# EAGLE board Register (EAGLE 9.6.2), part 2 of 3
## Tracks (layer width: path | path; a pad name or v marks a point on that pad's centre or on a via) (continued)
GND  (via drill 0.35) (continued)
  Bottom 0.152: 30.47,60.25 30.47,61.49 C82.2 30.47,61.67 30.47,73.23 C77.2 30.47,73.41 30.47,84.96 C75.2 31.91,85.09 32.07,85.25 32.07,87.78 30.47,89.38 30.47,96.16 C10.2 30.47,96.34 30.47,107.54 C53.2 30.65,107.72 30.65,108.79 | 30.47,60.25 v34.02,60.25 37.22,63.45 43.27,63.45 | 30.65,109.14 30.65,115.19 GND.1 | 30.65,109.14 30.65,108.79 | 30.65,109.14 v32.07,109.14 | 30.47,16.51 30.47,27.89 C48.2 | C74.2 18.73,27.89 C14.2 18.73,28.07 18.73,39.27 C18.2 18.73,39.45 C65.2 18.73,50.65 18.73,61.85 C60.2 18.73,62.03 18.73,65.88 19.84,66.99 19.84,71.12 18.73,72.23 18.73,73.23 C55.2 18.55,73.41 18.55,78.34 16.95,79.94 16.95,84.96 C11.2 16.78,85.14 16.78,96.16 C69.2 16.95,96.34 16.95,102.39 17.13,102.57 17.13,106.48 | 30.47,16.51 29.4,15.44 v21.76,15.44 20.33,15.44 19.27,16.51 C74.2 | 30.47,16.51 C28.2 | C74.2 | 17.13,106.48 10.95,106.48 9.48,107.95 C9.2 8.06,108.08 8.15,107.99 8.15,100.53 7,99.38 7,96.88 C1.2 7,96.7 7,85.5 C3.2 7,85.32 7,74.12 C5.2 7,73.94 7,62.56 C7.2 | 17.13,106.48 17.49,106.48 18.55,107.54 C19.2 | v4.69,109.64 5.52,110.47 17.23,110.47 18.73,108.98 C19.2 | 7,62.33 7,62.38 C7.2 | 7,62.33 7,61.85 | 7,61.85 7,51.18 C2.2 7,51 7,39.8 C4.2 7,39.62 7,28.42 C6.2 7,28.25 7,26.66 | 7,26.66 7,16.87 C8.2 | 7,26.66 v9.89,26.66 | 7,62.33 v9.85,62.33 | 7,61.85 C7.2 | 30.65,108.79 27.44,108.79 26.38,107.72 18.73,107.72 C19.2 | C70.2 68.34,107.54 68.34,96.34 C76.2 68.34,96.16 68.34,85.14 C80.2 68.34,84.96 68.34,73.41 C86.2 68.34,73.23 68.34,61.67 C64.2 68.34,61.49 68.34,52.43 68.52,52.25 68.52,50.65 C26.2 68.52,50.47 68.52,39.62 68.34,39.45 C31.2 68.34,39.27 68.34,28.07 C16.2 68.34,27.89 68.34,26.82
  Bottom 0.152: 68.34,15.27 68.34,17.04 C68.2 68.34,17.22 68.34,26.82 | 68.34,15.27 68.34,6.73 C35.2 68.34,6.55 68.34,6.02 69.23,5.13 71.18,5.13 | 76.34,6.91 74.56,5.13 71.18,5.13 | 76.34,6.91 77.23,7.8 79.54,7.8 80.61,6.73 C36.2 | 68.34,15.27 v72.07,15.27 | 71.18,5.13 v71.18,5.31 | 45.05,75.18 45.05,84.96 C78.2 45.05,85.14 45.05,90.65 | 45.05,75.18 45.05,73.41 C87.2 | C49.2 45.22,107.54 45.22,96.34 C32.2 45.05,96.16 45.05,95.09 46.67,93.47 46.67,92.28 45.05,90.65 | 56.78,90.65 56.78,85.14 C79.2 56.78,84.96 56.78,73.41 C81.2 56.78,73.23 56.78,61.67 C63.2 56.78,61.49 v56.78,55.98 56.78,51.89 | 56.78,90.65 56.78,94.74 | 56.78,94.74 56.78,96.16 C54.2 56.78,96.34 56.78,100.97 | 56.78,100.97 56.78,107.54 C71.2 56.78,107.72 56.6,107.9 v56.6,108.97 | 56.78,100.97 v56.96,100.97 | 56.78,90.65 45.05,90.65 | 56.78,94.74 v56.6,94.74 | C43.2 44.34,6.73 43.98,7.09 43.98,16.69 C22.2 43.98,16.87 43.98,21.13 45.05,22.2 | C52.2 45.05,39.27 45.05,28.07 C41.2 45.05,27.89 45.05,22.2 | 56.78,51.89 56.78,50.65 C47.2 56.96,50.47 v56.96,49.05 56.96,41.05 v57.14,40.87 57.14,39.62 56.96,39.45 C30.2 56.78,39.27 56.78,28.07 C40.2 | 56.78,51.89 v56.6,51.89 | C44.2 56.07,6.73 55.36,7.44 55.36,16.69 C17.2 55.18,16.87 55.18,21.67 | 55.18,21.67 55.18,25.76 56.78,27.36 | 56.78,27.36 56.78,27.89 C40.2 | 45.05,22.2 47.18,22.2 47.71,21.67 55.18,21.67 | 68.34,26.82 57.32,26.82 56.78,27.36 | 56.78,27.36 C40.2 | 43.27,63.45 43.27,69.14 47.18,73.05 47.18,74.83 46.82,75.18 45.05,75.18
H0  (via drill 0.35)
  Top 0.152: v101.41,21.84 102.12,21.13 102.12,20.24 IC90.12 | v102.3,68.43 102.3,70.21 IC48.3
  Route2 0.152: v101.41,21.84 103.54,21.84 107.63,25.93 107.63,63.09 v102.3,68.43
H1  (via drill 0.35)
  Top 0.152: v76.16,27.36 75.27,26.47 75.27,23.62 75.45,23.44 76.34,23.44 78.3,21.49 78.3,20.24 IC93.12 | v100.52,71.98 103.09,71.98 103.37,71.71 103.37,70.38 IC48.4
  Route2 0.152: v78.65,66.29 86.12,66.29 90.62,70.8 99.33,70.8 v100.52,71.98
  Bottom 0.152: v76.16,27.36 76.16,63.81 v78.65,66.29
H2  (via drill 0.35)
  Top 0.152: v77.94,11.71 78.3,11.35 78.3,9.75 IC96.12 | v104.97,78.03 104.97,76.61 IC48.10
  Route14 0.152: v77.94,11.71 81.67,11.71 85.41,15.44 87.54,15.44 100.52,28.42 100.52,57.94 104.79,62.2 104.79,77.85 v104.97,78.03
H3  (via drill 0.35)
  Top 0.152: v100.34,21.84 99.45,21.84 97.32,19.71 97.32,13.84 95.9,12.42 92.34,12.42 90.21,10.29 90.21,9.75 IC99.12 | v101.22,74.24 101.25,74.21 102.34,74.21 103.37,75.24 103.37,76.25 IC48.11
  Route3 0.152: v100.34,21.84 100.34,28.78 100.52,28.96 100.52,58.11 98.21,60.43 98.21,73.03 99.18,73.99 99.9,73.99 100.15,74.24 v101.22,74.24
I0  (via drill 0.35)
  Top 0.152: v87.01,16.51 88.79,14.73 88.79,14.2 IC91.2 | v67.27,56.69 66.21,57.76 66.21,58.47 IC53.3
  Route14 0.152: v87.01,16.51 87.01,33.05 68.52,51.54 68.52,55.45 v67.27,56.69
I1  (via drill 0.35)
  Top 0.152: v69.58,18.29 68.34,18.29 64.78,14.73 64.78,14.2 IC94.2 | v69.76,56.69 68.52,56.69 67.45,57.76 67.45,58.47 IC53.4
  Bottom 0.152: v69.58,18.29 69.58,21.67 69.05,22.2 69.05,26.82 69.58,27.36 69.58,51.18 69.94,51.54 69.94,56.52 v69.76,56.69
I2  (via drill 0.35)
  Top 0.152: v64.96,6.38 64.78,6.2 64.78,3.71 IC97.2 | v77.41,50.29 75.45,52.25 75.27,52.25 71.89,55.63 71.89,65.76 71.18,66.47 69.23,66.47 68.69,65.94 68.69,64.69 IC53.10
  Route15 0.152: v64.96,6.38 64.96,7.09 75.81,17.93 75.81,18.64 92.88,35.71 92.88,38.38 82.92,48.34 79.36,48.34 v77.41,50.29
I3  (via drill 0.35)
  Top 0.152: v72.25,67.18 72.61,67.54 106.74,67.54 110.12,64.16 110.12,3.53 108.17,1.58 102.48,1.58 101.05,3 101.05,3.53 IC100.2 | v67.63,66.29 67.63,64.87 67.45,64.69 IC53.11
  Route2 0.152: v72.25,67.18 68.52,67.18 v67.63,66.29
J0  (via drill 0.35)
  Top 0.152: v95.9,21.84 95.9,12.95 95.72,12.78 90.92,12.78 90.21,13.49 90.21,14.02 IC91.3 | v101.59,60.07 101.9,60.07 102.23,59.74 IC58.3
  Bottom 0.152: v95.9,21.84 95.9,25.58 96.79,26.47 96.79,33.05 98.03,34.29 98.03,35.71 96.43,37.31 96.43,54.92 v101.59,60.07
J1  (via drill 0.35)
  Top 0.152: v75.81,16.33 75.45,16.69 68.16,16.69 66.21,14.73 66.21,14.2 IC94.3 | v100.34,60.07 101.05,60.78 102.26,60.78 103.37,59.68 103.37,58.65 IC58.4
  Route14 0.152: v75.81,16.33 86.12,16.33 86.65,15.8 87.36,15.8 91.1,19.53 91.1,50.83 v100.34,60.07
J2  (via drill 0.35)
  Top 0.152: v66.56,5.31 66.21,4.95 66.21,3.71 IC97.3 | v105.5,66.29 105.22,66.29 104.79,65.86 104.79,64.69 IC58.10
  Route2 0.152: v66.56,5.31 69.05,5.31 69.76,4.6 86.47,4.6 103.37,21.49 103.72,21.49 109.05,26.82 109.05,62.74 v105.5,66.29
J3  (via drill 0.35)
  Top 0.152: v106.92,60.78 109.77,57.94 109.77,3.71 107.99,1.93 103.37,1.93 102.3,3 102.3,3.53 IC100.3 | v103.54,62.92 103.54,64.52 IC58.11
  Route2 0.152: v106.92,60.78 105.68,60.78 v103.54,62.92
K0  (via drill 0.35)
  Top 0.152: v91.45,15.8 91.45,14.2 IC91.4 | v66.03,49.05 66.03,47.45 IC63.3
  Route3 0.152: v91.45,15.8 91.45,19.36 93.41,21.31 93.41,26.47 87.9,31.98 83.1,31.98 v66.03,49.05
K1  (via drill 0.35)
  Top 0.152: v74.56,15.44 71.89,12.78 67.98,12.78 67.45,13.31 67.45,14.02 IC94.4 | v67.45,49.05 67.45,47.45 IC63.4
  Route2 0.152: v74.21,49.4 67.81,49.4 v67.45,49.05
  Bottom 0.152: v74.56,15.44 74.56,17.76 74.21,18.11 74.21,35.53 74.92,36.25 74.92,48.69 v74.21,49.4
K2  (via drill 0.35)
  Top 0.152: v69.23,51.89 69.23,52.96 68.69,53.49 IC63.10 | IC97.4 67.31,2.54 66.67,1.91 62.71,1.91 v61.91,2.7
  Route14 0.152: v61.91,2.7 66.67,2.7 69.58,5.61 v69.58,5.84
  Bottom 0.152: v69.58,5.84 69.58,11.71 72.78,14.91 72.78,23.27 71.01,25.04 71.01,56.52 70.12,57.4 69.41,57.4 69.05,57.05 69.05,52.07 v69.23,51.89
K3  (via drill 0.35)
  Top 0.152: v103.54,5.31 103.54,3.71 IC100.4 | v67.81,51.89 67.81,53.14 67.45,53.49 IC63.11
  Route3 0.152: v103.54,5.31 103.54,8.15 107.45,12.07 107.45,13.49 99.63,21.31 99.63,23.62 79.54,43.71 76.52,43.71 69.05,51.18 68.52,51.18 v67.81,51.89
L0  (via drill 0.35)
  Top 0.152: v93.59,15.8 92.88,15.09 92.88,14.2 IC91.5 | v101.23,45.31 101.23,45.85 102.12,46.74 102.12,47.27 IC68.3
  Bottom 0.152: v93.59,15.8 93.59,17.22 98.39,22.02 98.39,35.89 96.79,37.49 96.79,40.87 v101.23,45.31
L1  (via drill 0.35)
  Top 0.152: v70.12,15.98 69.94,15.98 68.69,14.73 68.69,14.2 IC94.5 | v103.54,44.07 103.54,44.6 102.83,45.31 102.83,46.2 103.37,46.74 103.37,47.27 IC68.4
  Route14 0.152: v70.12,15.98 79.54,6.55 86.47,6.55 88.07,8.15 88.07,15.44 102.83,30.2 102.83,43.36 v103.54,44.07
L2  (via drill 0.35)
  Top 0.152: v74.92,6.55 69.23,6.55 68.69,6.02 68.69,3.71 IC97.5 | v105.14,55.27 105.14,54.03 104.79,53.67 IC68.10
  Route15 0.152: v74.92,6.55 79.18,6.55 104.61,31.98 105.68,31.98 106.21,32.51 106.21,54.2 v105.14,55.27
L3  (via drill 0.35)
  Top 0.152: v106.92,45.67 109.41,43.18 109.41,3.89 107.81,2.29 105.5,2.29 104.79,3 104.79,3.53 IC100.5 | v103.72,51.89 103.72,53.31 103.54,53.49 IC68.11
  Route2 0.152: v106.92,45.67 106.92,48.69 v103.72,51.89
M0  (via drill 0.35)
  Top 0.152: v67.63,34.11 66.21,35.53 66.21,36.25 IC73.3 | v92.34,21.84 92.88,21.84 93.94,20.78 93.94,20.24 IC91.9
  Route3 0.152: v67.63,34.11 80.07,34.11 v92.34,21.84
M1  (via drill 0.35)
  Top 0.152: v69.76,22.55 69.76,20.24 IC94.9 | v70.29,27.53 70.29,28.25 71.89,29.85 71.89,32.16 69.41,34.65 68.34,34.65 67.45,35.53 67.45,36.25 IC73.4
  Bottom 0.152: v69.76,22.55 69.76,25.93 69.58,26.11 69.58,26.82 v70.29,27.53
M2  (via drill 0.35)
  Top 0.152: v70.29,11.35 69.94,11 69.94,9.75 IC97.9 | v67.27,40.69 67.63,41.05 67.81,41.05 68.52,41.76 68.52,42.29 IC73.10
  Route2 0.152: v73.32,38.56 69.41,38.56 v67.27,40.69
  Bottom 0.152: v70.29,11.35 70.29,11.89 73.85,15.44 73.85,35.89 73.32,36.42 v73.32,38.56
M3  (via drill 0.35)
  Top 0.152: v67.45,44.07 67.45,42.47 IC73.11 | v106.74,12.42 106.74,11 106.21,10.47 106.21,9.75 IC100.9
  Route3 0.152: v67.45,44.07 67.45,46.56 65.32,48.69 65.32,49.4 65.67,49.76 69.94,49.76 87.36,32.33 90.39,32.33 99.28,23.44 99.28,19.89 v106.74,12.42
N0  (via drill 0.35)
  Top 0.152: v93.76,18.47 92.88,19.36 92.88,20.07 IC91.10 | IC78.3 102.23,34.99 v102.17,34.92
  Route2 0.152: v102.17,34.92 97.6,34.92 v97.32,34.65
  Bottom 0.152: v93.76,18.47 93.76,23.98 96.43,26.65 96.43,33.76 v97.32,34.65
N1  (via drill 0.35)
  Top 0.152: v63.89,32.69 63.36,32.69 62.12,31.45 62.12,24.87 60.69,23.44 60.69,17.4 61.05,17.04 66.03,17.04 68.52,19.53 68.52,20.07 IC94.10 | v102.1,33.95 102.74,33.95 103.37,34.58 103.37,36.25 IC78.4
  Route2 0.152: v63.89,32.69 91.99,32.69 93.23,33.93 102.08,33.93 v102.1,33.95
N2  (via drill 0.35)
  Top 0.152: v74.92,8.33 69.41,8.33 68.69,9.04 68.69,9.58 IC97.10 | v105.32,34.11 107.45,34.11 108.34,35 108.34,43.18 107.63,43.89 105.68,43.89 104.79,43 104.79,42.47 IC78.10
  Route15 0.152: v74.92,8.33 75.63,8.33 79.01,11.71 81.67,11.71 85.76,15.8 87.36,15.8 105.32,33.76 v105.32,34.11
N3  (via drill 0.35)
  Top 0.152: v105.68,12.42 104.79,11.53 104.79,9.75 IC100.10 | v106.92,44.6 105.14,44.6 103.54,43 103.54,42.47 IC78.11
  Bottom 0.152: v105.68,12.42 105.68,20.96 106.57,21.84 106.57,25.93 106.92,26.29 v106.92,44.6
N$1  (via drill 0.35)
  Top 0.152: IC9.3 4.69,104.88 4.69,105.09 4.74,105.15 v4.74,106.46 | v8.6,90.12 8.6,88.52 IC3.9 | v9.84,98.1 9.52,98.1 8.6,99.03 8.6,99.9 IC1.9 | v10.55,21.49 8.87,21.49 8.6,21.22 8.6,20.07 IC8.9 | v9.66,29.67 8.6,30.73 8.6,31.27 IC6.9 | v8.6,44.42 8.6,42.82 IC4.9 | v8.6,52.43 8.6,54.03 IC2.9 | v8.6,63.98 8.6,65.58 IC7.9 | v10.55,74.47 8.6,76.43 8.6,76.96 IC5.9
  Route2 0.152: v4.74,106.46 4.66,106.46 2.86,108.27 ADRESS.1
  Route15 0.152: v8.6,90.12 8.6,87.45 9.49,86.56 9.49,75.54 v10.55,74.47 | v9.84,98.1 9.84,108.26 2.91,115.19 ADRESS.1
  Bottom 0.152: v8.6,90.12 8.6,94.92 9.84,96.16 v9.84,98.1 | v10.55,21.49 10.55,28.78 v9.66,29.67 9.66,39.62 8.6,40.69 v8.6,44.42 9.31,45.14 9.31,51.18 8.6,51.89 v8.6,52.43 8.6,58.58 10.72,60.7 10.72,62.84 9.58,63.98 v8.6,63.98 10.55,65.94 v10.55,74.47
N$2  (via drill 0.35)
  Top 0.152: 2.22,74.05 0.97,75.3 0.97,89.88 3.44,92.35 3.44,93.68 IC1.2 3.44,93.85 3.44,95.45 1.49,97.41 1.49,100.97 3.44,102.92 3.44,104.88 IC9.2 | 2.22,74.05 3.44,72.83 3.44,70.92 IC5.2 | v3.44,80.7 3.44,82.3 IC3.2 | 2.22,74.05 v2.2,74.03 | v3.44,12.07 3.44,13.67 IC8.2 | v3.42,23.44 3.42,25.03 3.44,25.04 IC6.2 | v3.44,35.32 3.44,36.6 IC4.2 | v3.44,46.38 3.44,47.98 IC2.2 | v3.26,57.76 3.44,57.94 3.44,59.36 IC7.2 3.42,59.54 3.42,62.05 v3.26,62.2
  Bottom 0.152: v3.44,80.7 3.44,79.27 2.2,78.03 v2.2,74.03 2.2,63.27 v3.26,62.2 | v3.26,57.76 3.26,53.85 2.37,52.96 2.37,47.45 v3.44,46.38 3.44,41.34 2.93,40.83 2.93,39.01 3.44,38.49 v3.44,35.32 3.44,23.44 v3.42,23.44 2.22,22.24 2.22,13.28 v3.44,12.07
N$3  (via drill 0.35)
  Top 0.152: v4.91,15.2 4.91,14.42 4.86,14.38 4.86,13.84 IC8.3 | v8.2,18.13 7.68,18.13 7.3,18.51 IC8.10 | v8.6,28.25 5.75,28.25 4.86,27.36 4.86,25.22 IC6.3 | v8.42,29.67 7.35,30.73 7.35,31.27 IC6.10 | 7.18,40.69 4.86,38.38 4.86,36.78 IC4.3 | 7.18,40.69 7.18,42.65 IC4.10 | v4.86,46.38 4.86,47.98 IC2.3 | v4.33,55.8 6.29,55.8 7.18,54.92 7.18,54.2 IC2.10 | IC9.5 v7.3,106.2 | 7.18,40.69 7.21,40.69 8.28,39.62 v8.6,39.62
  Route14 0.152: ADRESS.2 5.4,108.11 v7.3,106.2 5.71,104.62 3.81,104.62 1.43,102.23 1.43,60.64 4.33,57.74 v4.33,55.8 5.87,54.26 5.87,47.39 v4.86,46.38 8.6,42.65 v8.6,39.62 8.6,29.85 v8.42,29.67 8.42,28.42 v8.6,28.25 8.54,28.19 8.54,18.47 v8.2,18.13 8.2,14.8 7.82,14.41 5.38,14.41 4.91,14.88 v4.91,15.2
N$4  (via drill 0.35)
  Top 0.152: IC7.3 4.69,59.54 4.69,60.66 v4.38,60.96 | IC5.3 4.69,70.74 4.69,67.72 v4.33,67.36 | v7.71,67.36 7.35,67 7.35,65.76 IC7.10 | v4.33,75.36 5.04,74.65 6.29,74.65 7.18,75.54 7.18,76.96 IC5.10 | 5.58,85.5 7.18,87.1 7.18,88.34 IC3.10 7.18,88.52 7.18,90.08 4.86,92.39 4.86,93.68 IC1.3 4.86,93.85 4.86,94.92 6.11,96.16 v8.24,96.16 | 5.58,85.5 4.86,84.79 4.86,82.47 IC3.3 | v7.71,98.3 7.35,98.65 7.35,99.9 IC1.10 | v6.06,106.16 6.11,106.11 6.11,104.88 IC9.4 | 5.58,85.5 v4.33,86.74
  Route2 0.152: v4.33,67.36 v7.71,67.36 | v8.24,96.16 7.71,96.7 v7.71,98.3 7.71,104.51 v6.06,106.16
  Route3 0.152: v4.38,60.96 4.33,61.01 v4.33,67.36 v4.33,75.36 4.33,75.47 4.63,75.77 4.63,86.44 v4.33,86.74
N$5  (via drill 0.35)
  Top 0.152: v7.18,15.44 6.11,14.38 6.11,13.84 IC8.4 | v6.1,18.41 6.11,18.42 6.11,19.89 IC8.11 | v10.91,36.07 10.91,35.89 10.2,35.18 6.82,35.18 6.11,35.89 6.11,36.6 IC4.4 | v6.11,41.05 6.11,42.65 IC4.11 | v9.18,106.97 9.84,106.3 IC9.7 9.84,103.55 10.33,103.07 11.12,103.07 v12.87,101.32 | v6.11,61.14 6.11,59.54 IC7.4 | v6.11,63.98 6.11,65.58 IC7.11 6.11,65.76 6.11,66.83 v8.06,68.78 | v10.2,80.16 7.71,80.16 6.11,81.76 6.11,82.3 IC3.4 | v6.07,89.96 5.93,89.82 5.93,88.52 IC3.11
  Route2 0.152: v6.11,41.05 10.91,36.25 v10.91,36.07 | v6.11,63.98 v6.11,61.14 | v6.07,89.96 6.07,87.49 10.2,83.36 v10.2,80.16
  Route3 0.152: v9.18,106.97 9.08,106.97 7.94,108.11 ADRESS.3 | v6.1,18.41 10.91,23.22 v10.91,36.07
  Route14 0.152: v7.18,15.44 6.1,16.52 v6.1,18.41
  Route15 0.152: v6.11,41.05 6.11,45.49 6.64,46.03 6.64,60.6 v6.11,61.14
  Bottom 0.152: v8.06,68.78 8.78,69.49 8.78,73.76 10.2,75.18 v10.2,80.16 10.2,80.52 12.87,83.19 v12.87,101.32
N$6  (via drill 0.35)
  Top 0.152: v6.12,92.39 6.12,93.13 6.11,93.14 6.11,93.68 IC1.4 | v8.93,97.62 8.9,97.59 6.88,97.59 6.11,98.36 6.11,99.9 IC1.11 | v8.95,102.74 8.6,103.1 8.6,104.88 IC9.6 | v11.62,28.78 10.38,27.53 7.09,27.53 6.11,26.55 6.11,25.22 IC6.4 | v11.62,30.91 11.62,31.45 10.06,33.01 6.66,33.01 6.11,32.45 6.11,31.45 IC6.11 | v7.71,49.76 7.18,49.76 6.11,48.69 6.11,48.16 IC2.4 | IC2.11 6.11,54.03 6.11,53.31 v8.24,51.18 v10.02,51.18 | v5.93,68.96 5.93,70.74 IC5.4 | IC5.11 6.09,76.99 v6.09,75.52
  Route2 0.152: v5.93,68.96 6.09,69.12 v6.09,75.52 | v6.12,92.39 8.93,95.21 v8.93,97.62 8.93,102.72 v8.95,102.74
  Route3 0.152: v5.93,68.96 5.93,65.23 7.71,63.45 7.71,51.71 v8.24,51.18
  Route15 0.152: v6.12,92.39 6.98,91.54 6.98,76.41 v6.09,75.52
  Bottom 0.152: v11.62,28.78 v11.62,30.91 11.62,49.58 v10.02,51.18 | v7.71,49.76 8.24,50.29 v8.24,51.18
N$7  (via drill 0.35)
  Top 0.152: v4.87,21.49 4.87,21.08 4.86,21.08 4.86,20.07 IC8.12 4.69,19.89 4.69,19 v3.98,18.29 | v7.89,23.58 7.3,24.17 IC6.5 | v7.18,12.07 7.18,13.67 IC8.5 | 2.73,40.16 3.62,41.05 4.15,41.05 4.69,41.58 4.69,42.65 IC4.12 | 2.73,40.16 1.49,38.91 1.49,30.2 2.3,29.39 4.13,29.39 4.69,29.94 4.69,31.27 IC6.12 4.86,31.45 4.86,31.98 6.64,33.76 v7.89,33.76 | v7.89,38.2 7.35,37.67 7.35,36.78 IC4.5 | ADRESS.4 10.55,115.19 11.09,114.66 11.09,111.1 IC9.9 11.11,109.67 12.15,108.62 v12.15,105.77 | v7.71,78.74 5.93,78.74 4.86,77.67 4.86,77.14 IC5.12 | v8.06,72.7 8.06,72.16 7.35,71.45 7.35,70.92 IC5.5 7.18,70.74 7.18,69.14 4.86,66.83 4.86,65.76 IC7.12 4.86,65.58 4.86,64.16 7.18,61.85 7.18,59.54 IC7.5 7.18,59.36 7.18,58.03 6.19,57.05 3.26,57.05 1.49,55.27 1.49,41.4 2.73,40.16
  Route14 0.152: v4.87,21.49 6.97,23.58 v7.89,23.58
  Route15 0.152: v7.89,23.58 7.89,27.39 7.55,27.72 7.55,33.42 v7.89,33.76
  Bottom 0.152: v7.18,12.07 5.98,12.07 3.98,14.07 v3.98,18.29 | v7.89,33.76 v7.89,38.2 | v8.06,72.7 8.06,74.83 7.71,75.18 v7.71,78.74 12.15,83.19 v12.15,105.77
N$8  (via drill 0.35)
  Top 0.152: v4.75,52.63 4.69,52.69 4.69,54.03 IC2.12 | v5.93,46.38 6.29,46.38 7.18,47.27 7.18,47.98 IC2.5 | v5.75,86.74 4.86,87.63 4.86,88.34 IC3.12 | v6.11,84.07 6.9,84.07 7.18,83.8 7.18,83.72 | IC3.5 7.27,82.37 7.18,82.46 7.18,83.72 | v10.55,102.03 8.6,102.03 8.42,102.21 5.04,102.21 4.69,101.85 4.69,100.08 IC1.12 | v10.55,96.16 10.55,96.14 9.67,95.26 7.75,95.26 7.35,94.86 7.35,94.39 | 7.35,94.39 7.35,93.85 IC1.5 | IC9.10 9.84,108.85 v10.55,108.14 | 7.18,83.72 10.55,87.1 10.55,89.59 8.78,91.36 8.1,91.36 7.3,92.16 IC1.5 | 7.35,94.39 IC1.5
  Route2 0.152: v5.75,86.74 5.75,84.43 v6.11,84.07 | v10.55,102.03 v10.55,108.14
  Route15 0.152: v6.11,84.07 5.22,83.19 5.22,53.14 4.75,52.67 v4.75,52.63 5.93,51.45 v5.93,46.38
  Bottom 0.152: v10.55,96.16 v10.55,102.03
N$9  (via drill 0.35)
  Top 0.152: IC88.5 104.79,24.87 104.79,27.53 107.28,30.02 107.28,30.91 IC88.8 107.45,31.09 108.17,31.8 v108.34,31.8 | v21.04,17.93 19.36,17.93 19.09,18.21 19.09,19.53 IC32.10 | v101.05,23.27 100.7,23.27 99.81,24.16 99.81,24.87 IC88.1 | v101.05,27.18 101.05,29.37 101.11,29.37 102.12,30.38 102.12,30.91 IC88.12 102.3,31.09 102.3,32.1 | v108.34,33.22 105.85,33.22 105.68,33.4 103.6,33.4 102.3,32.1 | v102.08,32.7 102.3,32.48 102.3,32.1
  Route2 0.152: v21.04,17.93 22.64,17.93 22.82,17.76 25.13,17.76 33.13,25.76 41.14,25.76 45.05,29.67 50.74,29.67 53.05,31.98 97.14,31.98 v97.5,32.33
  Route15 0.152: v97.5,32.33 97.87,32.7 v102.08,32.7
  Bottom 0.152: v101.05,27.18 v101.05,23.27 | v108.34,33.22 v108.34,31.8
N$10  (via drill 0.35)
  Top 0.152: v16.61,14.93 16.61,14.03 16.6,14.02 16.6,13.49 IC32.3 | v59.8,34.65 63.54,34.65 65.85,32.33 | 65.85,32.33 66.03,32.16 66.03,31.09 IC83.12 66.03,30.91 66.03,30.38 64.96,29.31 | 64.96,29.31 63.54,27.89 63.54,24.87 IC83.1 | 64.96,29.31 68.52,25.76 68.52,24.87 IC83.5 | 65.85,32.33 70.29,32.33 71.01,31.62 71.01,31.09 IC83.8
  Route3 0.152: v16.61,14.93 20.17,14.93 22.47,17.22 28.87,17.22 51.09,39.45 55,39.45 v59.8,34.65
N$11  (via drill 0.35)
  Top 0.152: v21.93,27.36 19.09,30.2 19.09,30.91 IC29.10 | v98.03,37.85 99.63,36.25 IC78.1 99.69,37.38 100.34,38.02 103.54,38.02 104.61,36.96 104.61,36.42 IC78.5 104.79,36.25 104.79,35.4 105.18,35 107.81,35 107.99,35.18 107.99,39.55 107.3,40.25 107.3,42.42 IC78.8 | v101.23,39.98 102.12,40.87 102.12,42.29 IC78.12
  Route2 0.152: v21.93,27.36 23,27.36 23.71,26.65 37.22,26.65 47.54,36.96 73.49,36.96 73.85,37.31 97.5,37.31 v98.03,37.85
  Bottom 0.152: v101.23,39.98 99.99,39.98 98.03,38.02 v98.03,37.85
N$12  (via drill 0.35)
  Top 0.152: v16.52,23.43 16.6,23.5 16.6,24.87 IC29.3 | 61.05,38.73 v53.05,38.73 | 62.47,37.31 63.36,36.42 IC73.1 | 62.47,37.31 61.05,38.73 | v65.49,44.07 66.03,43.54 66.03,42.47 IC73.12 | 61.05,38.73 v61.23,38.91 | 62.47,37.31 64.43,39.27 66.21,39.27 68.52,36.96 68.52,36.42 IC73.5 68.69,36.25 68.69,35.53 69.23,35 70.47,35 70.47,37.49 71.01,38.02 71.01,42.29 IC73.8
  Route14 0.152: v16.52,23.43 17.32,22.63 21.29,22.63 25.3,26.65 38.82,26.65 50.91,38.73 v53.05,38.73
  Bottom 0.152: v65.49,44.07 61.23,39.8 v61.23,38.91
N$13  (via drill 0.35)
  Top 0.152: v90.03,106.3 90.03,104.7 IC16.3 | v89.85,108.43 91.27,109.86 91.27,110.57 IC16.13 | v17.84,94.74 17.84,93.14 IC15.11 | v35.8,113.94 35.8,113.96 38.27,116.43 73.32,116.43 74.38,115.37 74.38,111.51 v74.45,111.44 | IC12.13 79.54,110.57 79.54,110.03 78.12,108.61 v78.12,108.26 | v78.3,106.3 78.3,104.7 IC12.3
  Route2 0.152: v17.84,94.74 17.84,95.99 v35.8,113.94
  Route3 0.152: v74.45,111.44 76.36,111.44 78.12,109.68 v78.12,108.26
  Route15 0.152: v89.85,108.43 88.43,108.43 87.72,107.72 78.65,107.72 v78.12,108.26
  Bottom 0.152: v90.03,106.3 90.03,108.26 v89.85,108.43 | v78.3,106.3 78.3,108.08 v78.12,108.26
N$14  (via drill 0.35)
  Top 0.152: v25.31,106.3 26.2,105.41 26.2,104.7 IC117.2 | v31.53,112.88 36.36,112.88 38.68,115.2 55.04,115.2 57.67,112.57 57.67,110.74 IC11.11
  Route2 0.152: v25.31,106.3 25.31,106.66 v31.53,112.88
N$15
  Top 0.152: IC117.4 29.04,104.52 29.04,103.81 31.18,101.68 42.02,101.68 42.38,101.32 45.76,101.32 47.54,103.1 55.54,103.1 56.43,103.99 56.43,104.52 IC11.5
N$16  (via drill 0.35)
  Top 0.152: v31.48,103.07 31.53,103.13 31.53,104.52 IC117.6 | IC10.11 46.04,109.6 v45.94,109.5
  Route3 0.152: v45.94,109.5 39.51,103.07 v31.48,103.07
N$17
  Top 0.152: IC10.5 44.69,104.7 44.69,105.23 42.02,107.9 34.02,107.9 32.78,109.14 32.78,110.57 IC117.10
N$18  (via drill 0.35)
  Top 0.152: 66.21,108.08 66.21,107.54 68.52,105.23 68.52,104.7 IC14.5 | 66.21,108.08 66.21,110.57 IC14.12 66.21,110.74 66.21,111.45 66.92,112.17 68.1,113.35 70.33,113.35 71.01,112.67 71.01,111.45 71.01,111.12 71.01,110.74 IC14.8 | v21.58,97.59 19.52,97.59 19.09,98.02 19.09,99.19 IC15.3 | v49.31,100.79 51.27,100.79 52.51,102.03 58.2,102.03 59.27,103.1 61.94,103.1 63.36,104.52 IC14.1 63.54,104.7 63.54,107.01 64.6,108.08 66.21,108.08
  Route3 0.152: v21.58,97.59 25.49,97.59 28.16,100.25 48.78,100.25 v49.31,100.79
N$19  (via drill 0.35)
  Top 0.152: IC28.8 107.28,99.37 107.28,99.9 106.57,100.61 103.01,100.61 102.3,99.9 102.3,99.37 IC28.12 102.12,99.19 102.12,98.12 v101.23,97.23 | v20.15,85.32 18.65,85.32 16.6,83.27 16.6,82.12 IC19.10 | v97.96,93.69 99.09,93.69 99.63,93.14 IC28.1 | IC28.5 104.77,91.13 v105.25,90.65
  Route2 0.152: v20.15,85.32 25.67,85.32 36.69,96.34 42.2,96.34 44.16,98.3 92.72,98.3 97.33,93.69 v97.96,93.69
  Route15 0.152: v105.25,90.65 104.37,89.76 v100.34,89.76
  Bottom 0.152: v100.34,89.76 100.34,90.83 97.94,93.24 97.94,94.47 97.96,94.49 | v97.96,93.69 97.96,94.49 | v101.23,97.23 100.7,97.23 97.96,94.49
N$20  (via drill 0.35)
  Top 0.152: 102.3,111.28 102.3,110.74 IC18.12 102.23,112.87 102.71,113.35 105.89,113.35 107.31,111.92 IC18.8 | 107.28,111.28 107.28,110.74 IC18.8 | v19.44,94.74 18.73,95.45 17.49,95.45 16.6,94.56 16.6,93.14 IC15.10 | v97.32,103.1 98.21,103.1 99.63,104.52 IC18.1 99.69,105.89 100.22,106.41 104.78,106.41 | 104.61,104.52 IC18.5 104.78,106.41 | IC18.8 107.28,110.57 107.28,108.92 104.78,106.41 | 104.78,106.41 104.72,106.36
  Route2 0.152: v19.44,94.74 20.51,94.74 21.93,96.16 27.62,96.16 34.56,103.1 v97.32,103.1
N$21  (via drill 0.35)
  Top 0.152: v53.94,94.74 53.94,93.14 IC21.3 | v53.94,97.59 54.29,97.94 54.47,97.94 55.18,98.65 55.18,99.19 IC21.13 | IC19.4 17.84,86.75 v17.83,86.73 | v33.49,100.97 42.38,100.97 43.45,99.9 43.45,99.37 IC20.13 | v42.2,94.74 42.2,93.14 IC20.3
  Route2 0.152: v33.49,100.97 33.49,100.81 19.42,86.73 v17.83,86.73
  Route15 0.152: v53.94,94.74 51.63,94.74 51.45,94.92 42.38,94.92 v42.2,94.74
  Bottom 0.152: v53.94,97.59 v53.94,94.74 | v42.2,94.74 40.07,96.88 37.58,96.88 v33.49,100.97
N$22  (via drill 0.35)
  Top 0.152: v40.6,106.66 39.71,105.77 39.71,104.7 IC10.1 | v64.96,107.37 64.78,107.19 64.78,104.7 IC14.2
  Route2 0.152: v64.96,107.37 64.96,109.68 70.47,115.19 JP16.1
  Bottom 0.152: v40.6,106.66 45.94,111.99 56.96,111.99 60.16,115.19 70.47,115.19 JP16.1
N$23
  Top 0.152: IC11.15 52.87,110.57 52.87,108.97 53.58,108.26 63.89,108.26 64.6,108.97 64.6,110.57 IC14.13 64.78,110.74 64.78,111.28 67.31,113.8 70.51,113.8 71.89,115.19 72.96,115.19 JP19.1
N$24  (via drill 0.35)
  Top 0.152: v51.45,106.3 51.45,104.7 IC11.1 | v69.83,112.54 69.94,112.43 69.94,110.57 IC14.9
  Bottom 0.152: v51.45,106.3 51.45,107.54 55.54,111.63 57.14,111.63 59.63,114.12 69.83,114.12 | 69.83,114.12 76.87,114.12 77.94,115.19 JP18.1 | 69.83,114.12 v69.83,112.54
N$25  (via drill 0.35)
  Top 0.152: IC10.15 40.96,111.28 v42.02,112.34 | v70.29,106.83 69.94,106.48 69.94,104.7 IC14.6
  Route2 0.152: v70.29,106.83 70.29,110.03 75.45,115.19 JP17.1
  Bottom 0.152: v42.02,112.34 56.78,112.34 60.87,116.43 74.38,116.43 JP17.1
N$26  (via drill 0.35)
  Top 0.152: v58.2,1.93 53.76,1.93 52.87,2.82 52.87,3.53 IC92.2 | v98.39,12.78 99.63,14.02 IC90.1
  Route2 0.152: v58.2,1.93 58.68,1.45 76.64,1.45 77.41,0.69 86.3,0.69 v98.39,12.78
N$27  (via drill 0.35)
  Top 0.152: 68.69,95.81 68.69,96.34 71.01,98.65 71.01,99.19 IC23.8 | 68.69,95.81 68.69,93.14 IC23.5 | v20.33,86.39 19.7,86.39 19.27,86.82 19.27,87.99 IC19.3 | v61.4,92.61 63,92.61 63.36,92.96 IC23.1 | v65.67,100.97 66.03,100.61 66.03,99.37 IC23.12 | v64.96,95.81 68.69,95.81
  Route3 0.152: v20.33,86.39 21.93,86.39 28.33,92.79 61.23,92.79 v61.4,92.61
  Bottom 0.152: v65.67,100.97 65.67,97.41 64.43,96.16 | 64.43,96.16 61.4,93.14 v61.4,92.61 | v64.96,95.81 64.6,96.16 64.43,96.16
N$28  (via drill 0.35)
  Top 0.152: IC68.12 102.3,53.67 102.3,55.09 103.19,55.98 105.5,55.98 107.28,54.2 107.28,53.67 IC68.8 107.28,53.49 107.28,52.25 103.9,48.87 | v22.47,43.89 19.98,43.89 19.09,43 19.09,42.47 IC27.10 | v88.43,49.76 97.32,49.76 99.28,47.8 | 99.28,47.8 99.63,47.45 IC68.1 | 103.9,48.87 104.61,48.16 104.61,47.45 IC68.5 | 103.9,48.87 100.34,48.87 99.28,47.8
  Route2 0.152: v22.47,43.89 28.87,43.89 29.22,43.54 52.7,43.54 56.08,46.91 61.04,46.91 66.74,52.6 85.59,52.6 v88.43,49.76
N$29  (via drill 0.35)
  Top 0.152: v44.34,78.38 43.98,78.74 40.25,78.74 35.45,73.94 34.56,73.94 31.53,70.92 31.53,70.38 IC114.6 | v57.49,86.56 57.49,87.99 57.67,88.16 IC31.11
  Route3 0.152: v44.34,78.38 45.58,78.38 46.82,79.63 48.78,79.63 55.71,86.56 v57.49,86.56
N$30  (via drill 0.35)
  Top 0.152: IC63.12 66.21,53.67 66.21,54.2 66.92,54.92 70.29,54.92 71.01,54.2 71.01,53.67 IC63.8 71.18,53.49 71.18,49.23 71.89,48.51 71.89,46.38 71.18,45.67 69.23,45.67 68.69,46.2 68.69,47.27 IC63.5 68.52,47.45 68.52,49.05 67.81,49.76 65.32,49.76 63.54,47.98 63.54,47.45 IC63.1 61.94,45.85 v61.05,45.85 | v22.47,39.98 21.93,39.45 19.09,39.45 16.6,36.96 16.6,36.42 IC27.3
  Route2 0.152: v22.47,39.98 25.67,39.98 28.87,43.18 53.94,43.18 56.6,45.85 v61.05,45.85
N$31
  Top 0.152: IC114.10 32.78,76.43 32.78,77.14 34.73,79.1 54.11,79.1 56.43,81.41 56.43,81.94 IC31.5
N$32  (via drill 0.35)
  Top 0.152: IC116.6 31.38,93.07 31.38,91.95 31.97,91.36 36.16,91.36 39.71,94.92 v39.89,94.92 | v81.32,113.06 92.16,113.06 93.94,111.28 93.94,110.74 IC16.11
  Route3 0.152: v39.89,94.92 40.25,94.92 45.22,99.9 60.87,99.9 74.03,113.06 v81.32,113.06
N$33  (via drill 0.35)
  Top 0.152: v39.71,97.59 33.85,97.59 32.78,98.65 32.78,99.19 IC116.10 | v59.63,102.39 66.56,102.39 67.27,101.68 71.18,101.68 v73.34,103.83 | IC16.5 92.7,104.52 92.7,103.99 92.08,103.37 v92.08,102.39
  Route2 0.152: v39.71,97.59 40.78,97.59 45.58,102.39 v59.63,102.39
  Route3 0.152: v92.08,102.39 74.77,102.39 v73.34,103.83
N$34  (via drill 0.35)
  Top 0.152: v27.98,97.59 29.04,97.59 30.11,98.65 30.11,99.19 IC116.12 | v79.54,113.77 81.14,112.17 81.32,112.17 82.21,111.28 82.21,110.74 IC12.11
  Route2 0.152: v27.98,97.59 27.98,100.97 31.53,104.52 58.03,104.52 69.94,116.43 75.98,116.43 77.05,115.37 77.05,114.83 78.12,113.77 v79.54,113.77
N$35  (via drill 0.35)
  Top 0.152: v29.76,101.68 28.16,101.68 26.38,99.9 26.38,99.37 IC116.15 | v69.58,107.54 78.65,107.54 80.96,105.23 IC12.5
  Route2 0.152: v29.76,101.68 32.6,101.68 35.09,104.17 66.21,104.17 v69.58,107.54
N$36  (via drill 0.35)
  Top 0.152: 38.65,109.32 38.29,109.32 37.93,109.68 37.93,112.01 40.28,114.36 53.37,114.36 55.18,112.55 55.18,110.74 IC11.13 55.18,110.57 55.18,110.03 54.47,109.32 54.29,109.32 v53.94,108.97 | 38.65,109.32 42.74,109.32 43.45,110.03 43.45,110.57 IC10.13 | v53.94,106.3 53.94,104.7 IC11.3 | v22.29,96.88 18.35,96.88 17.84,97.38 17.84,99.19 IC15.4 | v34.91,105.23 37.22,105.23 39.36,103.1 41.31,103.1 42.2,103.99 42.2,104.52 IC10.3 | v38.65,108.97 38.65,109.32
  Route2 0.152: v22.29,96.88 23.36,96.88 31.71,105.23 v34.91,105.23
  Bottom 0.152: v53.94,108.97 v53.94,106.3 | v34.91,105.23 v38.65,108.97
N$37  (via drill 0.35)
  Top 0.152: 80.43,28.96 80.43,29.31 79.72,30.02 79.72,30.91 IC85.13 | 80.43,28.96 80.78,28.6 v88.96,28.6 89.67,28.6 91.27,30.2 91.27,30.91 IC86.13 | IC86.3 90.19,24.89 90.19,26.05 89.6,26.65 v88.96,26.65 | v21.04,16.87 19.02,16.87 17.84,18.05 17.84,19.53 IC32.11 | v77.76,26.47 77.76,25.4 78.3,24.87 IC85.3 | 80.43,28.96 80.07,28.96 79.72,28.6 77.94,28.6 v77.76,28.78
  Route2 0.152: v21.04,16.87 29.76,16.87 32.25,14.38 48.43,14.38 55.36,21.31 72.61,21.31 v77.76,26.47
  Bottom 0.152: v88.96,28.6 v88.96,26.65 | v77.76,26.47 v77.76,28.78
N$38  (via drill 0.35)
  Top 0.152: IC81.13 55.18,30.91 55.18,30.38 54.11,29.31 54.11,24.87 IC81.3 53.94,24.87 53.94,24.33 53.05,23.44 v49.49,23.44 | v17.84,11.71 17.84,13.31 IC32.4 | v34.73,16.15 34.73,17.93 36.93,20.12 36.93,23.86 39.36,26.29 41.31,26.29 42.19,27.16 | 42.19,27.16 42.2,27.15 42.2,24.87 IC80.3 | 42.19,27.16 43.45,28.42 43.45,30.91 IC80.13
  Route3 0.152: v49.49,23.44 47.18,23.44 39.89,16.15 v34.73,16.15
  Bottom 0.152: v17.84,11.71 30.29,11.71 v34.73,16.15
N$39  (via drill 0.35)
  Top 0.152: v90.21,38.2 90.21,36.42 IC76.3 | v89.85,40.34 91.27,41.76 91.27,42.29 IC76.13 | v21.4,26.47 17.84,30.02 17.84,30.91 IC29.11 | v74.21,36.6 75.27,37.67 76.87,37.67 | 76.87,37.67 77.58,37.67 78.3,36.96 78.3,36.42 IC75.3 | 77.23,39.27 76.87,38.91 76.87,37.67 | 77.23,39.27 79.54,41.58 79.54,42.29 IC75.13 | 77.23,39.27 v77.05,39.45
  Route2 0.152: v21.4,26.47 23.36,26.47 23.53,26.29 38.47,26.29 48.78,36.6 v74.21,36.6 | v89.85,40.34 78.3,40.34 77.41,39.45 v77.05,39.45
  Bottom 0.152: v90.21,38.2 90.21,38.73 89.85,39.09 v89.85,40.34
N$40
  Top 0.152: IC12.1 75.98,104.52 75.98,103.81 77.41,102.39 88.27,102.39 89.21,101.44 93.03,101.44 93.98,102.39 99.28,102.39 100.88,103.99 100.88,104.52 IC18.2
N$41
  Top 0.152: IC16.15 88.96,110.57 88.96,108.26 89.5,107.72 99.45,107.72 100.88,109.14 100.88,110.57 IC18.13
N$42
  Top 0.152: IC16.1 87.72,104.7 87.72,105.23 89.85,107.37 104.08,107.37 106.03,109.32 106.03,110.57 IC18.9
N$43
  Top 0.152: IC12.15 77.23,110.74 77.23,112.52 79.18,114.48 106.5,114.48 107.99,112.99 107.99,107.01 106.21,105.23 106.21,104.7 IC18.6
N$44
  Top 0.152: IC98.2 40.96,3 43.09,0.86 73.14,0.86 75.81,3.53 IC96.1
N$45  (via drill 0.35)
  Top 0.152: IC114.12 30.29,76.43 30.29,77.14 31.27,78.12 v31.27,79.38 | IC30.11 46.04,86.56 v45.97,86.49
  Route3 0.152: v45.97,86.49 38.86,79.38 v31.27,79.38
N$46  (via drill 0.35)
  Top 0.152: v29.76,78.03 27.44,78.03 26.38,76.96 26.38,76.43 IC114.15 | v47.18,80.34 46.82,79.98 46.82,79.81 46.47,79.45 45.76,79.45 44.87,80.34 44.87,81.94 IC30.5
  Route2 0.152: v29.76,78.03 31,78.03 34.2,81.23 46.29,81.23 v47.18,80.34
N$47  (via drill 0.35)
  Top 0.152: v89.85,94.74 90.03,94.56 90.03,93.14 IC26.3 | v89.85,96.88 90.49,96.88 91.43,97.82 IC26.13 | IC19.11 17.84,80.72 v17.78,80.66 | IC25.3 78.3,92.96 78.3,92.43 77.58,91.72 75.1,91.72 74.38,92.43 v72.61,92.43 71.89,91.72 70.65,91.72 70.47,91.9 70.47,94.39 71.01,94.92 75.98,94.92 79.54,98.48 79.54,99.19 IC25.13
  Route3 0.152: v17.78,80.66 21.01,80.66 31,90.65 65.67,90.65 67.45,92.43 v72.61,92.43
  Route15 0.152: v89.85,94.74 88.79,94.74 87.72,93.68 73.85,93.68 v72.61,92.43
  Bottom 0.152: v89.85,96.88 v89.85,94.74
N$48  (via drill 0.35)
  Top 0.152: v53.94,83.72 53.94,82.12 IC31.3 | v54.47,86.56 55.18,87.27 55.18,88.16 IC31.13 | v23,69.67 21.49,68.17 18.4,68.17 17.84,68.72 17.84,70.21 IC13.4 | v34.73,80.52 41.31,80.52 42.2,81.41 42.2,81.94 IC30.3 42.38,82.12 42.38,84.43 43.45,85.5 43.45,88.16 IC30.13
  Route2 0.152: v23,69.67 25.13,71.81 25.13,72.34 25.67,72.87 26.38,72.87 34.02,80.52 v34.73,80.52
  Route15 0.152: v53.94,83.72 42.74,83.72 39.54,80.52 v34.73,80.52
  Bottom 0.152: v53.94,83.72 53.94,86.03 v54.47,86.56
N$49  (via drill 0.35)
  Top 0.152: 104.79,61.14 104.79,61.49 107.28,63.98 107.28,64.52 IC58.8 | 104.79,61.14 104.79,58.65 IC58.5 | v19.44,55.27 19.09,54.92 19.09,53.67 IC24.10 | v90.03,60.25 92.7,60.25 93.41,60.96 97.32,60.96 98.21,60.07 | 98.21,60.07 99.63,58.65 IC58.1 | v100.34,62.2 101.45,62.2 102.12,62.87 102.12,64.52 IC58.12 | 98.21,60.07 v98.92,60.78 99.28,61.14 104.79,61.14
  Route15 0.152: v19.44,55.27 20.69,55.27 20.87,55.09 33.31,55.09 36.51,58.29 88.07,58.29 v90.03,60.25
  Bottom 0.152: v98.92,60.78 v100.34,62.2
N$50  (via drill 0.35)
  Top 0.152: v30.24,86.75 30.24,87.5 30.29,87.45 30.29,88.16 IC115.12 | v48.07,96.16 53.4,96.16 54.11,96.88 55.89,96.88 57.67,98.65 57.67,99.19 IC21.11
  Route2 0.152: v30.24,86.75 30.24,86.84 32.55,89.14 32.55,90.33 38.21,95.99 47.89,95.99 v48.07,96.16
N$51  (via drill 0.35)
  Top 0.152: v40.7,91.36 39.99,90.65 27.22,90.65 26.38,89.81 26.38,88.16 IC115.15 | v49.49,92.08 50.74,92.08 51.09,91.72 55.71,91.72 56.43,92.43 56.43,92.96 IC21.5
  Route2 0.152: v40.7,91.36 42.04,92.71 48.86,92.71 v49.49,92.08
N$52
  Top 0.152: IC116.2 26.38,93.14 26.38,93.68 29.04,96.34 44.34,96.34 45.94,97.94 45.94,99.19 IC20.11
N$53  (via drill 0.35)
  Top 0.152: IC116.4 28.89,92.11 29.99,91.01 37.58,91.01 v38.65,92.08 | v44.78,91.68 44.69,91.77 44.69,92.96 IC20.5
  Route14 0.152: v38.65,92.08 44.39,92.08 v44.78,91.68
N$54  (via drill 0.35)
  Top 0.152: 71.01,88.16 71.01,88.88 70.29,89.59 69.41,89.59 69.23,89.41 69.23,86.92 68.16,85.85 67.27,85.85 66.21,86.92 66.21,88.16 IC33.12 | v23,68.61 22.05,67.65 17.98,67.65 16.6,69.04 16.6,70.21 IC13.3 | v60.34,80.34 61.76,80.34 63.36,81.94 IC33.1 63.54,82.12 63.54,82.65 64.25,83.36 67.81,83.36 | 67.81,83.36 68.52,82.65 68.52,82.12 IC33.5 | 71.01,88.16 71.01,86.56 67.81,83.36 | 71.01,88.16 IC33.8
  Route2 0.152: v23,68.61 25.84,68.61 36.69,79.45 59.45,79.45 v60.34,80.34
N$55  (via drill 0.35)
  Top 0.152: 107.28,88.16 107.28,88.7 106.39,89.59 103.01,89.59 102.3,88.88 102.3,88.16 IC38.12 | v19.44,78.03 19.09,77.67 19.09,76.43 IC13.10 | v89.85,84.25 93.59,84.25 93.76,84.43 97.32,84.43 99.45,82.3 | 99.45,82.3 99.63,82.12 IC38.1 99.45,82.3 | 104.61,83.78 104.61,83.66 104.61,82.12 IC38.5 | 104.55,83.84 104.61,83.78 | 99.45,82.3 100.52,83.36 104.08,83.36 104.55,83.84 | 107.28,88.16 107.28,86.56 104.65,83.94 104.61,83.9 | 104.55,83.84 104.61,83.9 | 107.28,88.16 IC38.8 | 104.61,83.78 104.61,83.9
  Route2 0.152: v19.44,78.03 28.69,78.03 35.8,85.14 87.36,85.14 88.25,84.25 v89.85,84.25
N$56  (via drill 0.35)
  Top 0.152: v19.8,60.6 17.19,60.6 16.6,60.01 16.6,59 IC17.3 | v48.96,67.36 53.99,67.36 54.76,68.13 62.87,68.13 63.5,68.76 IC43.1 63.5,71.36 63.18,71.67 v63.18,72.52 63.36,72.7 66.74,72.7 67.45,71.98 | v65.67,78.03 66.03,77.67 66.03,76.43 IC43.12 | 67.45,71.98 68.52,70.92 68.52,70.38 IC43.5 | 67.45,71.98 71.01,75.54 71.01,76.25 IC43.8
  Route2 0.152: v19.8,60.6 27.98,60.6 34.73,67.36 v48.96,67.36
  Bottom 0.152: v65.67,78.03 65.67,76.61 63.18,74.12 v63.18,72.52
N$57  (via drill 0.35)
  Top 0.152: v20.51,74.65 18.91,74.65 17.84,75.72 17.84,76.25 IC13.11 | IC35.3 78.3,81.94 78.12,81.76 v78.12,80.34 78.83,79.63 88.07,79.63 | 88.07,79.63 88.43,79.63 90.03,81.23 90.03,81.94 IC36.3 | v78.12,85.85 79.54,87.27 79.54,88.16 IC35.13 | v88.07,85.5 88.43,85.85 89.67,85.85 91.27,87.45 91.27,88.16 IC36.13 | 88.07,79.63 v88.07,79.98
  Route15 0.152: v20.51,74.65 23.18,77.32 75.1,77.32 v78.12,80.34
  Bottom 0.152: v78.12,80.34 v78.12,85.85 | v88.07,79.98 v88.07,85.5
N$58  (via drill 0.35)
  Top 0.152: v41.14,94.74 40.78,94.74 39.71,93.68 39.71,93.14 IC20.1 | v55,94.74 55.54,94.74 56.6,95.81 62.65,95.81 64.6,93.85 64.6,93.14 IC23.2
  Route2 0.152: v41.14,94.74 41.85,95.45 54.29,95.45 v55,94.74
N$59
  Top 0.152: IC21.15 52.87,99.37 52.87,100.08 54.47,101.68 63,101.68 64.6,100.08 64.6,99.37 IC23.13
N$60
  Top 0.152: IC21.1 51.45,93.14 51.45,93.68 54.29,96.52 68.16,96.52 69.76,98.12 69.76,99.19 IC23.9
N$61  (via drill 0.35)
  Top 0.152: v69.41,94.74 69.76,94.39 69.76,93.14 IC23.6 | v44.51,97.59 42.02,97.59 40.96,98.65 IC20.15
  Route2 0.152: v69.41,94.74 68.52,94.74 66.38,96.88 45.22,96.88 v44.51,97.59
N$62  (via drill 0.35)
  Top 0.152: v53.58,5.31 53.94,4.95 53.94,3.71 IC92.3 | v98.39,13.84 98.39,15.62 100.88,18.11 100.88,20.07 IC90.13
  Route2 0.152: v53.58,5.31 57.49,5.31 60.85,1.95 73.5,1.95 74.25,2.7 80.53,2.7 84.66,2.7 85.41,1.95 86.49,1.95 v98.39,13.84
N$63  (via drill 0.35)
  Top 0.152: 66.21,63.98 66.21,64.52 IC53.12 66.21,63.98 | v16.07,49.05 16.42,48.69 16.42,47.45 IC24.3 | v61.4,59 63,59 63.18,58.83 | 63.18,58.83 63.36,58.65 IC53.1 63.18,58.83 | 63.18,58.83 64.25,59.89 67.81,59.89 68.52,59.18 68.52,58.65 IC53.5 | v64.6,62.38 66.21,63.98 | v70.64,62.39 71.12,62.86 IC53.8
  Route2 0.152: v16.07,49.05 16.95,49.05 31.71,63.81 56.6,63.81 v61.4,59
  Route15 0.152: v64.6,62.38 v70.64,62.38 v70.64,62.39
  Bottom 0.152: v64.6,62.38 61.4,59.18 v61.4,59
N$64  (via drill 0.35)
  Top 0.152: v90.03,71.98 90.03,70.38 IC46.3 | v90.39,78.03 91.27,77.14 91.27,76.43 IC46.13 | v18.33,66.85 v18.31,66.85 17.84,66.38 17.84,65.05 IC17.11 | 70.47,67.89 71.54,67.89 72.25,68.61 72.25,68.96 75.27,71.98 77.76,71.98 78.3,71.45 78.3,70.38 IC45.3 | 70.47,67.89 v64.17,67.89 | 76.57,73.94 72.96,73.94 70.47,71.45 70.47,67.89 | 76.57,73.94 78.47,73.94 79.54,75.01 79.54,76.25 IC45.13 | 76.57,73.94 v76.57,74.65
  Route2 0.152: v90.39,78.03 89.32,78.03 86.65,75.36 77.29,75.36 v76.57,74.65
  Route15 0.152: v18.33,66.85 18.74,67.26 28.26,67.26 31.14,70.14 47.11,70.14 49.36,67.89 v64.17,67.89
  Bottom 0.152: v90.03,71.98 90.03,77.67 v90.39,78.03
N$65  (via drill 0.35)
  Top 0.152: v26.56,83.72 26.38,83.54 26.38,82.12 IC115.2 | v85.41,95.45 91.69,95.45 93.94,97.7 93.94,99.19 IC26.11
  Route2 0.152: v26.56,83.72 28.33,83.72 33.67,89.05 48.07,89.05 52.69,93.68 74.03,93.68 75.81,95.45 v85.41,95.45
N$66  (via drill 0.35)
  Top 0.152: v29.4,83.72 29.04,83.36 29.04,82.12 IC115.4 | v35.62,89.94 40.42,89.94 41.49,91.01 43.61,91.01 44.13,90.49 49.96,90.49 50.48,91.01 72.07,91.01 72.43,90.65 77.94,90.65 78.3,91.01 v89.38,91.01 | 92.88,93.14 IC26.5 v92.71,91.75 v92.71,91.74
  Route2 0.152: v89.38,91.01 90.11,91.74 v92.71,91.74
  Route3 0.152: v35.62,89.94 v29.4,83.72
N$67  (via drill 0.35)
  Top 0.152: v38.65,86.92 38.11,86.39 35.27,86.39 31.53,82.65 31.53,82.12 IC115.6 | v80.07,94.74 80.07,95.63 82.21,97.77 82.21,99.19 IC25.11
  Route2 0.152: v38.65,86.92 38.73,86.92 40.07,88.25 47.8,88.25 52.87,93.32 74.21,93.32 75.63,94.74 v80.07,94.74
N$68  (via drill 0.35)
  Top 0.152: v37.4,87.1 37.05,86.74 33.49,86.74 32.78,87.45 32.78,88.16 IC115.10 | v73.85,91.36 79.72,91.36 80.96,92.61 IC25.5
  Route2 0.152: v37.4,87.1 38.82,85.67 68.16,85.67 v73.85,91.36
N$69  (via drill 0.35)
  Top 0.152: 50.74,70.38 50.74,72.16 53.58,75.01 54.47,75.01 55.18,75.72 55.18,76.25 IC41.13 | 50.74,70.38 50.74,69.14 50.91,68.96 53.23,68.96 53.94,69.67 53.94,70.21 IC41.3 | v17.84,57.23 17.84,58.83 IC17.4 | v38.29,69.32 38.82,69.32 39.18,68.96 41.49,68.96 42.2,69.67 42.2,70.21 IC40.3 42.38,70.38 42.38,70.92 43.45,71.98 43.45,76.25 IC40.13 | v49.49,70.38 50.74,70.38
  Route2 0.152: v17.84,57.23 17.84,65.05 20.69,67.89 29.58,67.89 31,69.32 v38.29,69.32 39.36,70.38 v49.49,70.38
N$70  (via drill 0.35)
  Top 0.152: 102.3,76.43 IC48.12 102.23,77.38 v101.59,78.03 102.3,78.74 105.5,78.74 107.28,76.96 107.28,76.43 IC48.8 | v23,66.29 22.68,66.61 19.32,66.61 19.09,66.38 19.09,65.05 IC17.10 | v76.7,68.61 77.76,68.61 78.12,68.25 98.95,68.25 99.69,69 IC48.1 99.81,70.38 99.81,72.16 | 99.81,72.16 99.81,72.34 100.16,72.7 103.78,72.7 104.61,71.87 104.61,70.38 IC48.5 | 99.81,72.16 v99.45,72.16
  Route2 0.152: v23,66.29 28.51,66.29 30.82,68.61 68.69,68.61 69.41,69.32 75.98,69.32 v76.7,68.61
  Bottom 0.152: v101.59,78.03 101.59,77.67 98.92,75.01 98.92,72.7 v99.45,72.16
N$71  (via drill 0.35)
  Top 0.152: v15.35,105.82 15.35,104.7 IC34.2
  Route14 0.152: CLK.1 15.56,106.02 v15.35,105.82
N$72
  Top 0.152: IC34.1 13.93,104.7 13.93,108.08 13.04,108.97 13.04,115.19 W.1
N$73  (via drill 0.35)
  Top 0.152: v74.92,92.96 75.81,92.96 IC25.1 | v97.32,91.72 100.16,91.72 100.88,92.43 100.88,92.96 IC28.2
  Route2 0.152: v74.92,92.96 96.08,92.96 v97.32,91.72
N$74
  Top 0.152: IC26.15 88.96,99.37 88.96,99.9 90.03,100.97 99.81,100.97 100.88,99.9 100.88,99.37 IC28.13
N$75  (via drill 0.35)
  Top 0.152: v87.72,94.74 87.72,93.14 IC26.1 | v90.92,94.74 92.7,94.74 94.48,96.52 105.14,96.52 106.03,97.41 106.03,99.19 IC28.9
  Bottom 0.152: v87.72,94.74 88.79,94.74 89.5,94.03 90.21,94.03 v90.92,94.74
N$76  (via drill 0.35)
  Top 0.152: v100.34,95.81 103.9,95.81 106.03,93.68 106.03,93.14 IC28.6 | v88.79,96.88 88.09,96.88 85.72,99.24 85.72,100.11 84.56,101.28 77.98,101.28 77.23,100.53 77.23,99.37 IC25.15
  Route3 0.152: v100.34,95.81 96.43,95.81 96.08,96.16 89.5,96.16 v88.79,96.88
N$77  (via drill 0.35)
  Top 0.152: v52.69,5.84 52.87,6.02 53.94,6.02 55.18,4.78 55.18,3.71 IC92.4 | v84.34,5.66 84.34,8.15 86.65,10.47 86.65,13.13 87.54,14.02 IC91.1
  Bottom 0.152: v52.69,5.84 52.69,5.13 53.23,4.6 67.81,4.6 68.16,4.24 82.92,4.24 v84.34,5.66
N$83  (via drill 0.35)
  Top 0.152: v41.67,83.72 40.78,83.72 39.71,82.65 39.71,82.12 IC30.1 | v59.27,80.34 59.98,79.63 63,79.63 64.6,81.23 64.6,81.94 IC33.2
  Route2 0.152: v41.67,83.72 52.87,83.72 55.71,80.87 58.74,80.87 v59.27,80.34
N$84
  Top 0.152: IC31.15 52.87,88.16 52.87,88.88 53.94,89.94 63.54,89.94 64.6,88.88 64.6,88.16 IC33.13
N$85
  Top 0.152: IC31.1 51.45,82.12 51.45,82.65 54.29,85.5 68.34,85.5 69.76,86.92 69.76,88.16 IC33.9
N$86  (via drill 0.35)
  Top 0.152: v71.89,83.54 71.72,83.36 70.65,83.36 69.94,82.65 69.94,82.12 IC33.6 | IC30.15 v40.96,84.43
  Route2 0.152: v71.89,83.54 71.54,83.54 71.36,83.36 55.36,83.36 54.29,84.43 v40.96,84.43
N$87  (via drill 0.35)
  Top 0.152: v76.34,7.98 75.98,7.62 65.14,7.62 63.72,6.2 58.56,6.2 56.6,4.24 56.6,3.71 IC92.5 | v88.96,21.84 88.96,20.24 IC91.13
  Bottom 0.152: v76.34,7.98 76.34,9.04 88.96,21.67 v88.96,21.84
N$90  (via drill 0.35)
  Top 0.152: v31.18,67.18 30.29,66.29 30.29,64.69 IC113.12 | v90.92,89.76 92.88,89.76 93.94,88.7 93.94,88.16 IC36.11
  Route14 0.152: v31.18,67.18 31.18,68.25 40.25,77.32 52.87,77.32 64.43,88.88 90.03,88.88 v90.92,89.76
N$91  (via drill 0.35)
  Top 0.152: v29.58,66.29 27.44,66.29 26.38,65.23 26.38,64.69 IC113.15 | v89.85,79.98 91.27,79.98 92.7,81.41 92.7,81.94 IC36.5
  Route14 0.152: v29.58,66.29 33.67,66.29 34.91,67.54 48.07,67.54 53.76,73.23 56.07,73.23 59.8,76.96 86.12,76.96 89.14,79.98 v89.85,79.98
N$92  (via drill 0.35)
  Top 0.152: v26.38,73.94 26.2,73.76 26.2,70.38 IC114.2 | v73.14,89.59 77.41,89.59 78.3,90.48 80.96,90.48 82.21,89.23 82.21,88.16 IC35.11
  Route3 0.152: v26.38,73.94 38.82,73.94 54.47,89.59 v73.14,89.59
N$93  (via drill 0.35)
  Top 0.152: v31.89,67.89 30.65,67.89 29.04,69.49 29.04,70.21 IC114.4 | v80.61,80.34 80.61,81.59 80.96,81.94 IC35.5
  Route14 0.152: v31.89,67.89 45.94,67.89 55.36,77.32 77.58,77.32 v80.61,80.34
N$98
  Top 0.152: IC35.1 75.98,81.94 75.98,81.41 78.12,79.27 98.74,79.27 100.88,81.41 100.88,81.94 IC38.2
N$99
  Top 0.152: IC36.15 88.96,88.16 88.96,88.88 90.56,90.48 100.7,90.48 101.05,90.12 101.05,88.16 IC38.13
N$100
  Top 0.152: IC36.1 87.72,82.12 87.72,83.19 89.67,85.14 104.53,85.14 106.03,86.64 IC38.9
N$101  (via drill 0.35)
  Top 0.152: v80.61,89.76 78.12,89.76 77.23,88.88 77.23,88.16 IC35.15 | v99.99,79.45 101.23,79.45 101.41,79.27 103.9,79.27 106.03,81.41 106.03,81.94 IC38.6
  Route2 0.152: v80.61,89.76 89.67,89.76 v99.99,79.45
N$102
  Top 0.152: IC92.9 57.85,9.75 57.85,10.29 59.63,12.07 68.52,12.07 68.87,12.42 74.21,12.42 75.81,14.02 IC93.1
N$103  (via drill 0.35)
  Top 0.152: v18.02,26.47 17.84,26.29 17.84,24.87 IC29.4 | 37.89,33.93 39.43,33.93 39.87,34.37 41.33,34.37 42.2,35.24 42.2,36.25 IC70.3 | 37.89,33.93 v35.27,33.93 | v49.31,34.82 53.05,34.82 53.94,35.71 53.94,36.25 IC71.3 | v55.89,40.87 55.36,41.4 55.36,42.29 IC71.13 | IC70.13 43.5,41.28 42.58,40.36 41.87,40.36 41.2,39.69 39.37,39.69 37.89,38.21 37.89,33.93
  Route2 0.152: v18.02,26.47 19.98,26.47 27.44,33.93 v35.27,33.93
  Route15 0.152: v49.31,34.82 36.16,34.82 v35.27,33.93
  Bottom 0.152: v55.89,40.87 55.89,27 55.71,26.82 52.87,26.82 49.31,30.38 v49.31,34.82
N$104  (via drill 0.35)
  Top 0.152: v26.4,57.03 26.38,57.06 26.38,58.47 IC113.2 | v53.58,73.94 55.89,73.94 57.67,75.72 57.67,76.25 IC41.11
  Route3 0.152: v26.4,57.03 29.58,57.03 46.31,73.76 53.4,73.76 v53.58,73.94
N$105  (via drill 0.35)
  Top 0.152: IC113.4 28.89,60.17 31.61,62.9 39.73,62.9 v39.89,62.74 | v59.8,71.98 58.92,71.98 58.2,72.7 57.49,72.7 56.6,71.81 56.6,70.38 IC41.5
  Route3 0.152: v39.89,62.74 48.43,71.27 59.09,71.27 v59.8,71.98
N$106  (via drill 0.35)
  Top 0.152: IC113.6 31.38,58.58 31.38,60.27 v32.07,60.96 | v46.47,74.47 46.04,74.91 IC40.11
  Bottom 0.152: v32.07,60.96 34.2,60.96 45.4,72.16 45.76,72.16 46.47,72.87 v46.47,74.47
N$107
  Top 0.152: IC113.10 32.78,64.69 32.78,65.41 35.62,68.25 43.27,68.25 44.69,69.67 44.69,70.21 IC40.5
N$112  (via drill 0.35)
  Top 0.152: v42.38,71.98 40.78,71.98 39.71,70.92 39.71,70.38 IC40.1 | v64.71,71.67 64.6,71.56 64.6,70.38 IC43.2
  Route2 0.152: v42.38,71.98 43.09,71.27 64.31,71.27 v64.71,71.67
N$113
  Top 0.152: IC41.15 52.87,76.43 52.87,77.14 53.94,78.21 63.54,78.21 64.6,77.14 64.6,76.43 IC43.13
N$114
  Top 0.152: IC41.1 51.45,70.38 51.45,70.92 53.76,73.23 67.81,73.23 69.76,75.18 69.76,76.25 IC43.9
N$115  (via drill 0.35)
  Top 0.152: IC40.15 40.96,75.1 41.41,74.65 v42.2,74.65 | v69.05,71.98 69.05,71.63 69.76,70.92 69.76,70.38 IC43.6
  Route2 0.152: v42.2,74.65 45.22,74.65 46.65,73.23 67.81,73.23 v69.05,71.98
N$116  (via drill 0.35)
  Top 0.152: v62.65,8.33 57.32,8.33 56.6,9.04 56.6,9.58 IC92.10 | v74.92,18.47 75.98,18.47 77.05,19.53 77.05,20.07 IC93.13
  Route2 0.152: v62.65,8.33 64.07,8.33 74.21,18.47 v74.92,18.47
N$118  (via drill 0.35)
  Top 0.152: v53.94,60.25 53.94,58.65 IC51.3 | v53.94,62.92 54.29,63.27 54.47,63.27 55.18,63.98 55.18,64.52 IC51.13 | v18.02,49.05 17.84,48.87 17.84,47.45 IC24.4 | v41.31,56.87 42.2,57.76 42.2,58.47 IC50.3 42.38,58.65 42.38,59.18 43.45,60.25 48.6,60.25 49.49,59.36 v49.49,59 | v41.67,62.03 43.45,63.81 43.45,64.52 IC50.13
  Route2 0.152: v18.02,49.05 25.67,49.05 32.78,56.16 40.6,56.16 v41.31,56.87
  Bottom 0.152: v53.94,62.92 v53.94,60.25 50.74,60.25 v49.49,59 | v41.67,62.03 41.67,57.23 v41.31,56.87
N$119  (via drill 0.35)
  Top 0.152: v40.07,51.18 34.56,51.18 31.53,48.16 31.53,47.45 IC112.6 | v88.61,74.65 92.7,74.65 93.94,75.89 93.94,76.25 IC46.11
  Route14 0.152: v40.07,51.18 41.14,51.18 44.51,54.56 53.23,54.56 72.61,73.94 87.9,73.94 v88.61,74.65
N$120  (via drill 0.35)
  Top 0.152: v40.25,56.87 35.62,52.25 33.49,52.25 32.78,52.96 32.78,53.49 IC112.10 | v92.66,71.67 92.71,71.67 IC46.5
  Route14 0.152: v40.25,56.87 58.74,75.36 88.96,75.36 v92.66,71.67
N$121  (via drill 0.35)
  Top 0.152: v38.29,53.14 37.05,51.89 34.2,51.89 33.49,51.18 31,51.18 30.29,51.89 30.29,53.49 IC112.12 | IC45.11 82.23,74.71 v82.23,74.7
  Route3 0.152: v38.29,53.14 57.14,53.14 72.61,68.61 v72.96,68.61
  Route14 0.152: v72.87,72.23 72.96,72.14 v72.96,68.61
  Route15 0.152: v82.23,74.7 79.75,72.23 v72.87,72.23
N$122  (via drill 0.35)
  Top 0.152: v31.53,56.69 30.65,55.8 27.98,55.8 26.38,54.2 26.38,53.67 IC112.15 | v71.18,68.61 71.54,68.96 71.72,68.96 75.1,72.34 79.54,72.34 80.96,70.92 IC45.5
  Route3 0.152: v31.53,56.69 36.87,56.69 38.47,58.29 57.49,58.29 67.09,67.89 70.47,67.89 v71.18,68.61
N$127
  Top 0.152: IC45.1 75.98,70.21 75.98,68.25 76.34,67.89 99.89,67.89 100.88,68.88 100.88,70.21 IC48.2
N$128
  Top 0.152: IC46.15 88.96,76.43 88.96,77.67 90.03,78.74 99.81,78.74 100.88,77.67 100.88,76.43 IC48.13
N$129
  Top 0.152: IC46.1 87.72,70.38 87.72,70.92 90.39,73.58 103.72,73.58 106.03,75.89 106.03,76.25 IC48.9
N$130  (via drill 0.35)
  Top 0.152: v105.5,71.98 106.03,71.45 106.03,70.38 IC48.6 | v78.12,74.65 77.23,75.54 77.23,76.25 IC45.15
  Route2 0.152: v105.5,71.98 101.59,71.98 99.63,73.94 86.04,73.94 85.13,73.03 82.99,73.03 82.93,73.09 79.68,73.09 v78.12,74.65
N$131  (via drill 0.35)
  Top 0.152: v56.25,11.35 55.36,10.47 55.36,9.75 IC92.11 | v62.47,13.31 63.36,14.2 IC94.1
  Bottom 0.152: v56.25,11.35 60.52,11.35 v62.47,13.31
N$132  (via drill 0.35)
  Top 0.152: v31.18,45.31 30.29,44.42 30.29,42.47 IC111.12 | v55.89,63.09 55.89,65.94 56.07,66.12 56.96,66.12 57.67,65.41 57.67,64.69 IC51.11
  Route2 0.152: v31.18,45.31 31.71,45.31 48.6,62.2 55,62.2 v55.89,63.09
N$133  (via drill 0.35)
  Top 0.152: v53.58,11.35 53.94,11 53.94,9.75 IC92.12 | v61.4,17.76 62.83,17.76 64.6,19.53 64.6,20.07 IC94.13
  Route2 0.152: v53.58,11.35 55,11.35 v61.4,17.76
N$134  (via drill 0.35)
  Top 0.152: v29.58,44.25 27.62,44.25 26.38,43 26.38,42.47 IC111.15 | v55.89,60.07 55.89,59.18 56.43,58.65 IC51.5
  Route2 0.152: v29.58,44.25 34.2,44.25 44.51,54.56 50.38,54.56 v55.89,60.07
N$135  (via drill 0.35)
  Top 0.152: v29.58,51.89 26.38,48.69 26.38,47.45 IC112.2 | v34.56,55.27 40.6,61.32 43.27,61.32 45.94,63.98 45.94,64.52 IC50.11
  Route2 0.152: v29.58,51.89 30.29,51.89 33.67,55.27 v34.56,55.27
N$136
  Top 0.152: IC112.4 29.04,47.45 29.04,48.16 31.71,50.83 33.67,50.83 34.38,51.54 37.76,51.54 39,52.78 39,54.74 40.42,56.16 42.91,56.16 44.69,57.94 44.69,58.47 IC50.5
N$141
  Top 0.152: IC50.1 39.71,58.65 39.71,59.18 41.14,60.6 48.96,60.6 50.38,59.18 50.38,57.23 50.74,56.87 63.72,56.87 64.6,57.76 64.6,58.47 IC53.2
N$142
  Top 0.152: IC51.15 52.87,64.69 52.87,65.41 53.94,66.47 60.34,66.47 62.83,63.98 62.83,63.45 63,63.27 63.89,63.27 64.6,63.98 64.6,64.52 IC53.13
N$143
  Top 0.152: IC51.1 51.45,58.65 51.45,59.18 53.94,61.67 67.98,61.67 69.76,63.45 69.76,64.52 IC53.9
N$144  (via drill 0.35)
  Top 0.152: IC50.15 40.96,65.23 42.02,66.29 v44.69,66.29 | v60.87,60.6 68.34,60.6 69.76,59.18 69.76,58.65 IC53.6
  Route2 0.152: v44.69,66.29 55.18,66.29 v60.87,60.6
N$145  (via drill 0.35)
  Top 0.152: v43.27,1.93 42.38,2.82 42.38,3.53 IC98.3 | IC96.13 77.05,9.58 77.05,7.62 76.52,7.09 76.52,5.72 v76.56,5.67
  Route3 0.152: v76.56,5.67 76.56,3.22 v74.03,0.69
  Bottom 0.152: v43.27,1.93 43.8,1.93 45.05,0.69 v74.03,0.69
N$146  (via drill 0.35)
  Top 0.152: v48.25,2.29 44.16,2.29 43.62,2.82 43.62,3.53 IC98.4 | v60.34,3.53 63.36,3.53 IC97.1
  Bottom 0.152: v48.25,2.29 57.49,2.29 58.74,3.53 v60.34,3.53
N$147  (via drill 0.35)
